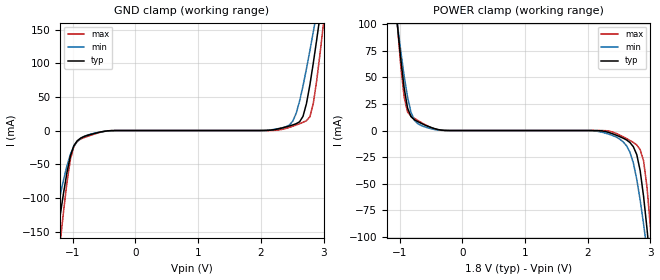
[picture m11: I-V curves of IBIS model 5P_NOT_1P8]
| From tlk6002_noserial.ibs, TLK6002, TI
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[Model]   5P_NOT_1P8
Model_type   Input
Polarity   Non-Inverting
Vinh =  1
Vinl =  0.8
C_comp   1.885425p   1.715283p   2.176444p
[Model Spec]
Vinh   1   0.955   1.045
Vinl   0.8   0.755   0.845
[Temperature Range]   25   125   -40
[Voltage Range]   1.8   1.71   1.89
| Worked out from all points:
|   GND clamp passes 1 mA (typ) near -0.48 V on its own axis
|   POWER clamp passes 1 mA (typ) near -0.39 V on its own axis
[POWER_clamp]
-1.8V     644.6mA    525mA      776.9mA
-1.036V   100.1mA    100.9mA    100.7mA
-872.7mV  21.16mA    31.46mA    17.46mA
-763.6mV  10.12mA    9.635mA    11.46mA
-490.9mV  2.713mA    1.555mA    2.652mA
2.182V    -152.1uA   -1.006mA   -8.499uA
2.727V    -15.22mA   -30.4mA    -11.16mA
2.836V    -37.78mA   -65.48mA   -18.08mA
2.945V    -92.52mA   -112.6mA   -53.32mA
3V        -126.4mA   -138.6mA   -91.27mA
3.055V    -162.4mA   -165.5mA   -136mA
3.545V    -523.2mA   -429.8mA   -609.7mA
[GND_clamp]
-1.8V     -566.4mA   -409.5mA   -760.6mA
-1.364V   -238.1mA   -175.1mA   -320.1mA
-1.255V   -162.4mA   -121.6mA   -216.8mA
-1.2V     -126.4mA   -96.48mA   -167.1mA
-1.036V   -37.78mA   -35.22mA   -42.81mA
-818.2mV  -8.811mA   -8.808mA   -10.5mA
2.4V      5.294mA    5.687mA    3.129mA
2.564V    10.12mA    25.72mA    8.206mA
2.727V    40.06mA    91.69mA    14.59mA
2.836V    100.1mA    146.6mA    40.3mA
3V        209mA      234.6mA    159.7mA
3.545V    604.1mA    545.7mA    644.5mA
